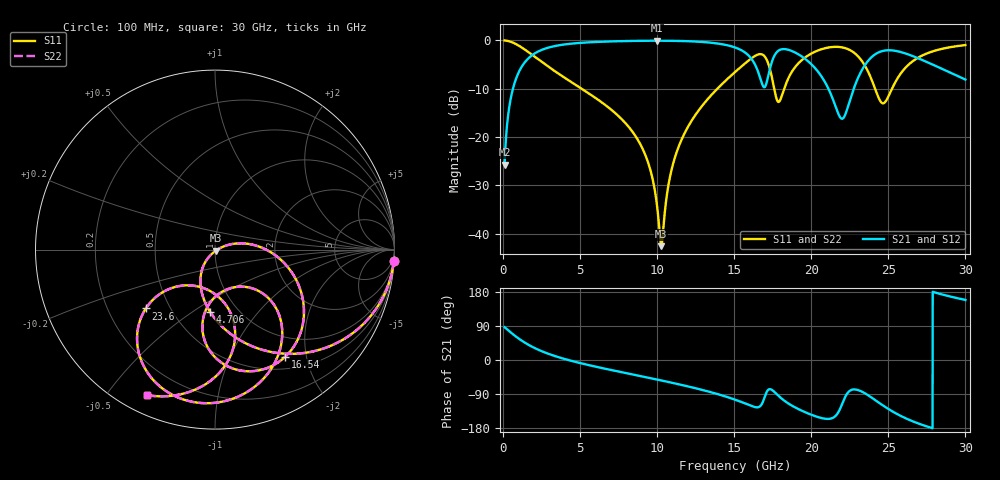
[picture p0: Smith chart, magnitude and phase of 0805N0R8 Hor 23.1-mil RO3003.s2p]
# GHz S MA R 50
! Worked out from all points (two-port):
!   3201 points, 100 MHz to 30 GHz, reference 50 ohm
!   highest |S21| = -0.07 dB at 9.995 GHz (marker M1); lowest = -25.7 dB at 100 MHz (marker M2)
!   |S21| within 3 dB of the highest: 1.882 GHz to 15.91 GHz (14.03 GHz wide, 158 % of centre); 24.06 GHz to 26.44 GHz (2.377 GHz wide, 9.41 % of centre)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
!   lowest |S11| = -42.5 dB at 10.27 GHz (marker M3), VSWR 1.02, Z = 50.4 - j0.632 ohm
!   |S11| at or under -10 dB: 5.101 GHz to 13.9 GHz (8.802 GHz wide, 92.6 % of centre); 17.6 GHz to 18.24 GHz (644.8 MHz wide, 3.6 % of centre); 24.14 GHz to 25.24 GHz (1.097 GHz wide, 4.44 % of centre)
!   |S22| runs from -42.5 to 0.0 dB; largest |S21 - S12| = 0
!   S11 on the Smith chart (normalised r, x): 100 MHz: 1, -32; 4.706 GHz: 0.75, -0.59; 16.54 GHz: 0.67, -1.64; 23.6 GHz: 0.37, -0.32; 30 GHz: 0.08, -0.64
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0.1  0.9986 -3.5  0.05195 86.5  0.05195 86.5  0.9986 -3.5
0.5298125  0.9639 -18.3  0.2659 71.7  0.2659 71.7  0.9639 -18.3
1.249281  0.8369 -39.9  0.5463 50.0  0.5463 50.0  0.8369 -39.9
2.762969  0.5605 -70.7  0.8258 19.1  0.8258 19.1  0.5605 -70.7
4.706469  0.3471 -94.6  0.9342 -5.1  0.9342 -5.1  0.3471 -94.6
5.089563  0.3171 -98.3  0.9446 -9.0  0.9446 -9.0  0.3171 -98.3
8.640187  0.09978 -126.8  0.9889 -40.1  0.9889 -40.1  0.09978 -126.8
9.995031  0.01933 -119.9  0.9924 -51.6  0.9924 -51.6  0.01933 -119.9
10.06978  0.01502 -113.5  0.9923 -52.2  0.9923 -52.2  0.01502 -113.5
10.266  0.007458 -57.2  0.9922 -53.9  0.9922 -53.9  0.007458 -57.2
10.85466  0.04049 19.2  0.9906 -59.1  0.9906 -59.1  0.04049 19.2
11.60216  0.09571 18.4  0.9855 -65.9  0.9855 -65.9  0.09571 18.4
15.05  0.4705 -19.1  0.8456 -104.6  0.8456 -104.6  0.4705 -19.1
16.53566  0.714 -56.9  0.4796 -124.7  0.4796 -124.7  0.714 -56.9
17.32053  0.5023 -96.9  0.5124 -76.9  0.5124 -76.9  0.5023 -96.9
17.88116  0.231 -69.8  0.7853 -94.9  0.7853 -94.9  0.231 -69.8
20.03956  0.7364 -65.0  0.5599 -145.0  0.5599 -145.0  0.7364 -65.0
21.99241  0.8475 -104.8  0.1547 -116.9  0.1547 -116.9  0.8475 -104.8
23.59953  0.5062 -139.6  0.5905 -90.8  0.5905 -90.8  0.5062 -139.6
25.01978  0.2667 -85.2  0.7912 -129.6  0.7912 -129.6  0.2667 -85.2
27.41178  0.7233 -91.2  0.6064 -174.1  0.6064 -174.1  0.7233 -91.2
30  0.8949 -114.9  0.3937 158.5  0.3937 158.5  0.8949 -114.9
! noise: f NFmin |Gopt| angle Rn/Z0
0.1  0.0015  0.9639  1.42  0.009387
3.417  0.007703  0.7519  19.82  0.00608
6.743  0.01331  0.725  36.76  0.008683
10.06  0.01997  0.7322  52.96  0.01198
13.39  0.03391  0.7895  68.5  0.02281
16.7  0.2907  0.9672  84.02  1.109
20.03  0.1498  0.927  98.26  0.1953
23.35  0.2873  0.9556  112.2  0.454
26.67  0.1432  0.9023  125.1  0.06895
30  0.1413  0.8914  137.2  0.0385
